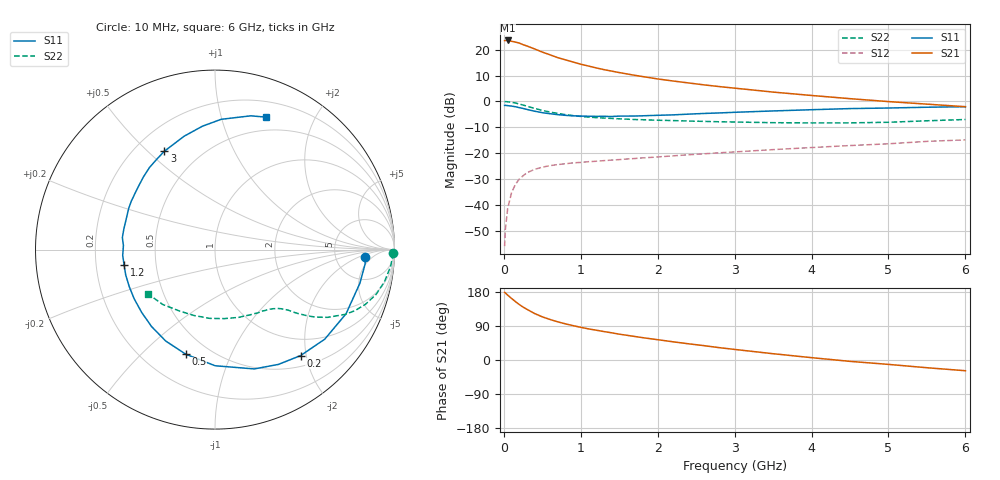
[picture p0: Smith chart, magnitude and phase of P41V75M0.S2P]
! SIEMENS Small Signal Semiconductors
! BFP182
! Si NPN RF Bipolar Junction Transistor in SOT143
! VCE = 1.75 V  IC = 5 mA
! Common Emitter S-Parameters:  March  1996
# GHz  S  MA  R  50
!  f  S11  S21  S12  S22
! GHz  MAG  ANG  MAG  ANG  MAG  ANG  MAG  ANG
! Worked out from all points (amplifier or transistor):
!   36 points, 10 MHz to 6 GHz, reference 50 ohm
!   highest |S21| = 23.5 dB at 50 MHz (marker M1)
!   |S21| within 3 dB of that: start of sweep to 376 MHz
!   unconditionally stable (mu >= 1): 1.556 GHz to 5.545 GHz
!   at 250 MHz: K = 0.22, MSG = 25.3 dB, |S12| = -28.7 dB
!   at 1.4 GHz: K = 0.95, MSG = 17.2 dB, |S12| = -22.7 dB
!   at 6 GHz: K = 0.96, MSG = 6.4 dB, |S12| = -14.9 dB
!   S11 on the Smith chart (normalised r, x): 10 MHz: 11, -3; 200 MHz: 0.68, -1.90; 500 MHz: 0.37, -0.69; 1.2 GHz: 0.32, -0.07; 3 GHz: 0.32, +0.56; 6 GHz: 0.35, +1.39
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0.01  0.8376 -2.8  14.94 178.5  0.0016 88.6  0.9904 -1.1
0.02  0.8404 -5.4  15.01 176.9  0.0034 83.6  0.9908 -2.2
0.05  0.8287 -13.1  15.04 171.1  0.0086 84.8  0.9826 -5.5
0.1  0.8129 -26.1  14.49 162.5  0.0172 75.8  0.9608 -10.8
0.15  0.7894 -39.2  14.01 154.2  0.0249 69.3  0.9311 -15.6
0.2  0.7589 -51.1  13.38 146.5  0.0315 64.2  0.8918 -20.0
0.25  0.7307 -61.1  12.47 139.7  0.0366 59.4  0.8504 -23.6
0.3  0.6998 -71.8  11.77 133.8  0.0419 54.7  0.8092 -26.5
0.4  0.6472 -89.9  10.32 122.6  0.0487 48.3  0.7329 -31.0
0.5  0.6052 -105.6  8.963 113.9  0.0536 43.2  0.6704 -34.1
0.6  0.5787 -118.3  7.945 106.9  0.0575 39.9  0.6232 -36.0
0.7  0.5556 -129.5  7.007 100.8  0.0603 37.4  0.5857 -37.5
0.9  0.5272 -148.6  5.761 90.7  0.065 35.2  0.5313 -39.5
1.1  0.5172 -164.1  4.824 82.1  0.0685 33.3  0.4982 -41.5
1.2  0.5135 -170.5  4.44 78.7  0.0699 32.7  0.4864 -42.5
1.7  0.5222 162.1  3.195 62.1  0.0789 32.3  0.4468 -48.1
2.2  0.5497 142.1  2.479 48.0  0.0888 31.9  0.4266 -55.5
3  0.6162 117.3  1.804 27.9  0.1058 30.3  0.4 -70.7
3.5  0.6545 105.3  1.514 16.6  0.1172 28.3  0.3882 -81.9
4.5  0.7267 87.3  1.13 -3.6  0.1404 23.6  0.3852 -107.5
5.5  0.7716 75.0  0.886 -20.4  0.1691 18.0  0.4225 -133.8
6  0.7906 69.0  0.79 -28.3  0.1808 13.8  0.4472 -146.5
